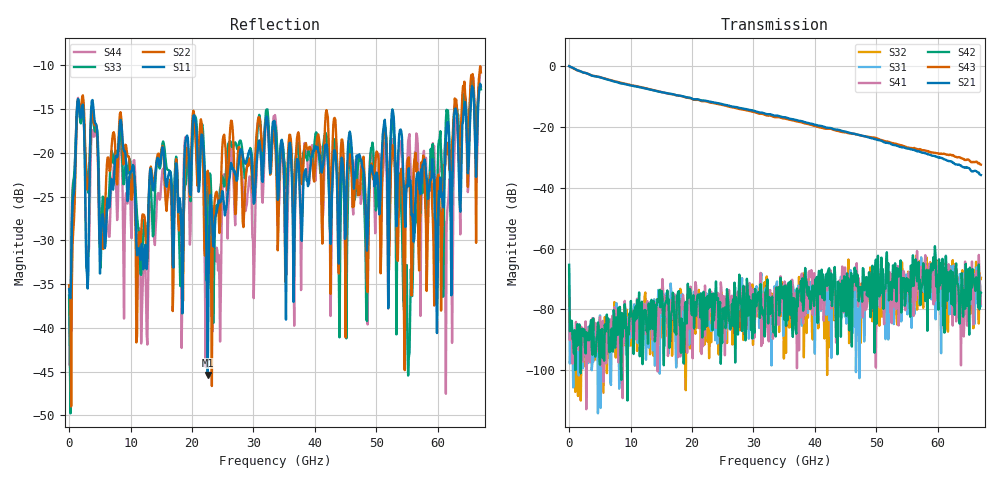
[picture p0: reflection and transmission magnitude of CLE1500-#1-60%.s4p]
!Keysight Technologies,N5247B,US50470101,A.16.20.02
!Date: Thursday, March 13, 2025 10:24:53
!Correction: S11(C  4-Port  )
!S12(C  4-Port  )
!S13(C  4-Port  )
!S14(C  4-Port  )
!S21(C  4-Port  )
!S22(C  4-Port  )
!S23(C  4-Port  )
!S24(C  4-Port  )
!S31(C  4-Port  )
!S32(C  4-Port  )
!S33(C  4-Port  )
!S34(C  4-Port  )
!S41(C  4-Port  )
!S42(C  4-Port  )
!S43(C  4-Port  )
!S44(C  4-Port  )
!S4P File: Measurements: <S11,S12,S13,S14>,
!<S21,S22,S23,S24>,
!<S31,S32,S33,S34>,
!<S41,S42,S43,S44>:
# Hz S  dB  R 50
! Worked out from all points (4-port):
!   601 points, 10 MHz to 67 GHz, reference 50 ohm
!   strongest paths, dB at 10 MHz, 16.76 GHz, 33.51 GHz, 50.25 GHz, 67 GHz:
!     S21: 0.0, -9.1, -16.3, -24.3, -35.8
!     S43: 0.0, -9.2, -16.8, -23.9, -32.4
!     S42: -65.4, -80.4, -86.0, -62.4, -74.5
!     S41: -75.7, -83.2, -73.0, -70.2, -78.2
!     S31: -66.9, -79.1, -79.9, -73.2, -78.9
!     S32: -72.6, -95.3, -79.0, -66.6, -69.6
!   lowest |S11| = -45.4 dB at 22.56 GHz (marker M1), VSWR 1.01, Z = 50 - j0.537 ohm
!   |S11| at or under -10 dB: start of sweep to end of sweep
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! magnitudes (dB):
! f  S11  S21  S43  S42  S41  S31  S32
! 10 MHz  -35.6  0.0  0.0  -65.4  -75.7  -66.9  -72.6
! 1.573 GHz  -14.1  -1.5  -1.5  -85.9  -93.4  -101.7  -92.8
! 22.56 GHz  -45.4  -11.5  -11.7  -75.6  -77.8  -78.1  -90.7
! 52.6 GHz  -15.0  -25.8  -25.3  -71.3  -73.9  -83.2  -82.1
! 55.39 GHz  -23.8  -27.2  -26.9  -74.9  -77.5  -71.4  -70.0
! 61.31 GHz  -18.3  -30.9  -29.0  -62.5  -69.6  -62.3  -64.4
! 67 GHz  -12.4  -35.8  -32.4  -74.5  -78.2  -78.9  -69.6
